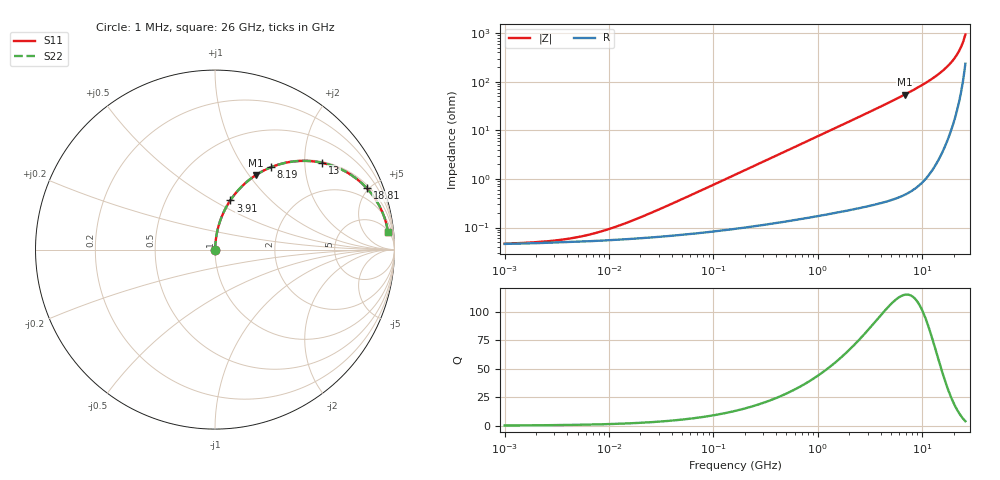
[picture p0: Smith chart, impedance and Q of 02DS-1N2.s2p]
# MHz S MA R 50
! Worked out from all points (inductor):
!   221 points, 1 MHz to 26 GHz, reference 50 ohm
!   read as one part in series: L = 1.2 nH near 25.4 MHz
!   highest Q = 115 at 6.808 GHz (marker M1), where L = 1.27 nH
!   S11 on the Smith chart (normalised r, x): 1 MHz: 1.00, +0.00; 3.91 GHz: 1.01, +0.60; 8.19 GHz: 1.01, +1.34; 13 GHz: 1.03, +2.45; 18.81 GHz: 1.19, +4.87; 26 GHz: 6, +18
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1  0.0004669 9.3  0.9995 -0.0  0.9995 -0.0  0.0004669 9.3
2.63894  0.0005255 22.2  0.9995 -0.0  0.9995 -0.0  0.0005255 22.2
5.52737  0.0006632 38.9  0.9995 -0.0  0.9995 -0.0  0.0006632 38.9
7.9995  0.0008064 48.3  0.9995 -0.0  0.9995 -0.0  0.0008064 48.3
11.5773  0.001036 57.3  0.9994 -0.0  0.9994 -0.0  0.001036 57.3
30.5518  0.002391 74.2  0.9994 -0.1  0.9994 -0.1  0.002391 74.2
168.871  0.01276 85.0  0.999 -0.7  0.999 -0.7  0.01276 85.0
425.516  0.03206 85.9  0.9982 -1.8  0.9982 -1.8  0.03206 85.9
891.261  0.06702 84.8  0.9961 -3.8  0.9961 -3.8  0.06702 84.8
1955.07  0.1462 80.7  0.987 -8.4  0.987 -8.4  0.1462 80.7
3910.05  0.2868 72.7  0.955 -16.7  0.955 -16.7  0.2868 72.7
4926.33  0.3561 68.6  0.9311 -20.9  0.9311 -20.9  0.3561 68.6
6807.69  0.4755 61.1  0.8756 -28.4  0.8756 -28.4  0.4755 61.1
8189.77  0.5548 55.8  0.8271 -33.7  0.8271 -33.7  0.5548 55.8
10318.4  0.6616 48.0  0.7432 -41.4  0.7432 -41.4  0.6616 48.0
13000.3  0.7695 38.9  0.6281 -50.3  0.6281 -50.3  0.7695 38.9
15639.6  0.8484 30.8  0.5115 -58.0  0.5115 -58.0  0.8484 30.8
18814.7  0.9128 22.0  0.3745 -65.8  0.3745 -65.8  0.9128 22.0
20636.4  0.9371 17.4  0.2997 -69.3  0.2997 -69.3  0.9371 17.4
22634.4  0.9552 12.8  0.222 -72.0  0.222 -72.0  0.9552 12.8
24825.9  0.9663 8.1  0.1427 -72.3  0.1427 -72.3  0.9663 8.1
26000  0.9692 5.7  0.1033 -69.8  0.1033 -69.8  0.9692 5.7
